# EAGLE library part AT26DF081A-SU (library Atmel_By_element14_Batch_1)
8-megabit Minimum SPI Serial Flash Memory
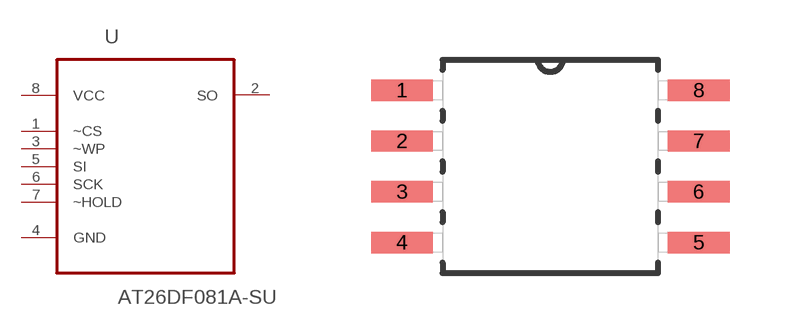
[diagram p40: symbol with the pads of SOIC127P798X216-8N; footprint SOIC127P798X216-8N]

Designator prefix U

## AT26DF081A-SU (MPN: AT26DF081A-SU; OC_FARNELL: 1455015; OC_NEWARK: -; PACKAGE: SOIC-8; SUPPLIER: Atmel)  [SOIC127P798X216-8N]
1  ~CS  in
2  SO  out
3  ~WP  in
4  GND  pas
5  SI  in
6  SCK  in
7  ~HOLD  in
8  VCC  pwr

## Footprint SOIC127P798X216-8N (pad centres in mm)
smd 1.549 x 0.533: 1 -3.708,1.905; 2 -3.708,0.635; 3 -3.708,-0.635; 4 -3.708,-1.905; 5 3.708,-1.905; 6 3.708,-0.635; 7 3.708,0.635; 8 3.708,1.905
